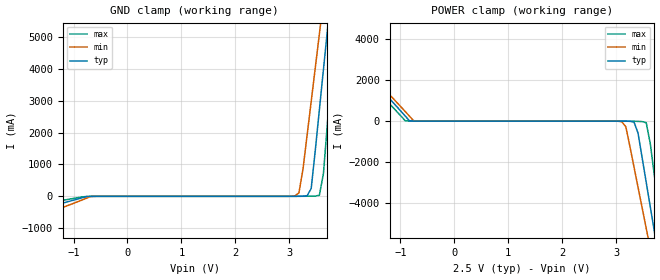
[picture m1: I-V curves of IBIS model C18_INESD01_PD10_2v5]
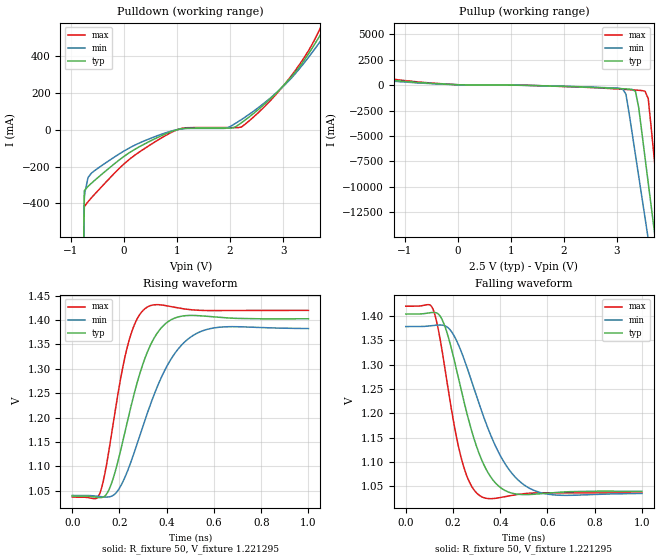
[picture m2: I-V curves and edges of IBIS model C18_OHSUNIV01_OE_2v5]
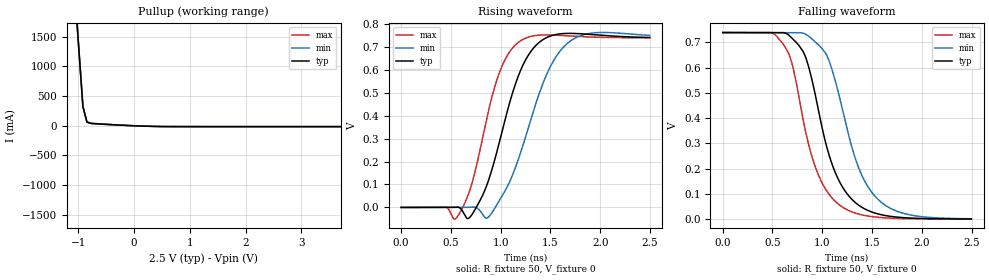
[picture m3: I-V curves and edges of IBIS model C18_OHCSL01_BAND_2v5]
|   This file is an IBIS representation of the   |
|   Integrated Device Technology, Inc.   |
|   ICS841N254I   |
|   FEMTOCLOCK NG CRYSTAL-TO-LVDS/HCSL CLOCK SYNTHESIZER   |
[IBIS Ver]   4.1
[File name]   841n254i.ibs
[File Rev]   1.0
[Date]   15 Mar 2010
[Source]   Originated at Integrated Device Technology, Inc.
[Disclaimer]
IDT hereby grants the user of this IBIS model a non-exclusive,
nontransferable license to use this IBIS model under the following terms.
Before using this IBIS model, the user should read this license.
If the user does not accept these terms,  the IBIS model should be
returned to IDT within 30 days.
   The user is granted this license only to use the IBIS model and
is not granted rights to sell, load, rent, lease or license the IBIS
model in whole or in part, or in modified form to anyone other than
user. User may modify the IBIS model to suit its specific
applications but rights to derivative works and such modifications
shall belong to IDT.
   This IBIS model is provided on an "AS IS" basis and IDT makes
absolutely no warranty with respect to the information contained
herein. IDT DISCLAIMS AND CUSTOMER WAIVES ALL WARRANTIES, EXPRESS
OR IMPLIED, INCLUDING WARRANTIES OF MERCHANTABILITY OR FITNESS FOR
A PARTICULAR PURPOSE. The entire risk as to quality and performance
is with the Customer. ACCORDINGLY, IN NO EVENT SHALL THE COMPANY BE
LIABLE FOR ANY DAMAGES, WHETHER IN CONTRACT OR TORT,INCLUDING ANY
LOST PROFITS OR OTHER INCIDENTAL, CONSEQUENTIAL, EXEMPLARY, OR
PUNITIVE DAMAGES ARISING OUT OF THE USE OR APPLICATION OF THE IBIS
model provided in this package. Further, IDT reserves the right to
make changes without notice to any product herein to improve
reliability, function, or design. IDT does not convey any license
under patent rights or any other intellectual property rights,
including those of third parties.
   IDT is not obligated to provide maintenance or support
for the licensed IBIS model.
[Copyright]   Copyright 2010 by Integrated Device Technology, Inc.
[Component]   ICS841N254KI
[Manufacturer] Integrated Device Technology, Inc.
[Package]
|LD QFN 32
|lead + wire   typ   min   max
R_pkg   72.4655m   58.886m   86.045m
L_pkg   1.47175nH   1.11650nH   1.77850nH
C_pkg   0.07747pF   0.07444pF   0.08050pF
[Pin] signal_name   model_name   R_pin   L_pin   C_pin
1   VDD   POWER   86.045m   1.77850nH   0.08050pF
2   NC   NC   76.996m   1.55783nH   0.07848pF
3   VDDA   POWER   67.941m   1.33717nH   0.07646pF
4   NC   NC   58.886m   1.11650nH   0.07444pF
5   GND   GND   58.886m   1.11650nH   0.07444pF
6   REF_CLK   C18_INESD01_PD10   67.941m   1.33717nH   0.07646pF
7   nOEA   C18_INESD01_PD10   76.996m   1.55783nH   0.07848pF
8   VDD   POWER   86.045m   1.77850nH   0.08050pF
9   nOEB   C18_INESD01_PD10   86.045m   1.77850nH   0.08050pF
10  REF_SEL   C18_INESD01_PD10   76.996m   1.55783nH   0.07848pF
11  XTAL_IN   NC   67.941m   1.33717nH   0.07646pF
12  XTAL_OUT   NC   58.886m   1.11650nH   0.07444pF
13  VDD   POWER   58.886m   1.11650nH   0.07444pF
14  BYPASS   C18_INESD01_PD10   67.941m   1.33717nH   0.07646pF
15  F_SEL0   C18_INESD01_PD10   76.996m   1.55783nH   0.07848pF
16  F_SEL1   C18_INESD01_PD10   86.045m   1.77850nH   0.08050pF
17  GND   GND   86.045m   1.77850nH   0.08050pF
18  QA1   C18_OHSUNIV01_OE   76.996m   1.55783nH   0.07848pF
19  nQA1   C18_OHSUNIV01_OE   67.941m   1.33717nH   0.07646pF
20  VDDOA   POWER   58.886m   1.11650nH   0.07444pF
21  QA0   C18_OHSUNIV01_OE   58.886m   1.11650nH   0.07444pF
22  nQA0   C18_OHSUNIV01_OE   67.941m   1.33717nH   0.07646pF
23  GND   GND   76.996m   1.55783nH   0.07848pF
24  IREF   NC   86.045m   1.77850nH   0.08050pF
25  GND   GND   86.045m   1.77850nH   0.08050pF
26  nQB1   C18_OHCSL01_BAND   76.996m   1.55783nH   0.07848pF
27  QB1   C18_OHCSL01_BAND   67.941m   1.33717nH   0.07646pF
28  VDDOB   POWER   58.886m   1.11650nH   0.07444pF
29  nQB0   C18_OHCSL01_BAND   58.886m   1.11650nH   0.07444pF
30  QB0   C18_OHCSL01_BAND   67.941m   1.33717nH   0.07646pF
31  GND   GND   76.996m   1.55783nH   0.07848pF
32  VDD   POWER   86.045m   1.77850nH   0.08050pF
[Diff Pin]  inv_pin  vdiff tdelay_typ tdelay_min  tdelay_max
18   19   NA   0   0   0
21   22   NA   0   0   0
27   26   NA   0   0   0
30   29   NA   0   0   0
[Model Selector] C18_INESD01_PD10
C18_INESD01_PD10_2v5  Buffer selection for 2v5
C18_INESD01_PD10_3v3  Buffer selection for 3v3
[Model Selector] C18_OHSUNIV01_OE
C18_OHSUNIV01_OE_2v5  Buffer selection for 2v5
C18_OHSUNIV01_OE_3v3  Buffer selection for 3v3
[Model Selector] C18_OHCSL01_BAND
C18_OHCSL01_BAND_2v5  Buffer selection for 2v5
C18_OHCSL01_BAND_3v3  Buffer selection for 3v3
| Models and submodels in the file (6): C18_INESD01_PD10_2v5 (Input), C18_OHSUNIV01_OE_2v5 (Output), C18_OHCSL01_BAND_2v5 (Open_source), C18_INESD01_PD10_3v3 (Input), C18_OHSUNIV01_OE_3v3 (Output), C18_OHCSL01_BAND_3v3 (Open_source)
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[Model] C18_INESD01_PD10_2v5
Model_type   Input
Polarity   Non-Inverting
Vinl = 0.7V
Vinh = 1.7V
|   typ   min   max
C_comp   2pF   1.5pF   2.5pF
|   typ   min   max
[Voltage range]   2.5V   2.375V   2.625V
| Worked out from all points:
|   GND clamp passes 1 mA (typ) near -0.63 V on its own axis
|   POWER clamp passes 1 mA (typ) near -0.64 V on its own axis
[GND_clamp]
|Voltage   I (typ)   I (min)   I (max)
-2.5V     -750.5mA   -1.114A    -470.1mA
-681.8mV  -2.012mA   -6.108mA   -2.703mA
3.106V    574.9uA    12.03mA    60.91uA
3.182V    1.627mA    109.8mA    268.6uA
3.258V    3.996mA    865.2mA    1.08mA
3.409V    245.5mA    2.979A     5.107mA
3.561V    2.713A     5.094A     32.39mA
3.636V    3.983A     6.152A     713.8mA
3.712V    5.254A     7.21A      2.338A
3.788V    6.512A     8.257A     3.947A
3.864V    7.757A     9.294A     5.539A
5V        25.01A     23.66A     27.6A
[Power_clamp]
|Voltage   I (typ)   I (min)   I (max)
-2.5V     4.507A     4.598A     4.173A
-833.3mV  19.22mA    247mA      7.107mA
-681.8mV  1.627mA    3.397mA    2.058mA
3.106V    -505.4uA   -25.77mA   -25.85uA
3.182V    -2.012mA   -269.5mA   -184.8uA
3.333V    -42.94mA   -2.236A    -4.112mA
3.409V    -586.1mA   -3.238A    -10.29mA
3.561V    -2.995A    -5.243A    -78.7mA
3.636V    -4.2A      -6.246A    -1.114A
3.712V    -5.406A    -7.249A    -2.656A
3.864V    -7.781A    -9.225A    -5.693A
5V        -24.15A    -22.85A    -26.63A
[Model] C18_OHSUNIV01_OE_2v5
Model_type   Output
Polarity   Non-Inverting
|   typ   min   max
C_comp   2pF   1.5pF   2.5pF
Vmeas = 1.22V
Rref = 50
Cref = 0
Vref = 1.22V
|   typ   min   max
[Voltage range]   2.5V   2.375V   2.625V
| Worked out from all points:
|   slope of the pulldown table from 0 to 0.375 V, typ, clamps not added: 5.71 ohm
|   slope of the pullup table from 0 to 0.375 V, typ, clamps not added: 13.8 ohm
|   rising waveform, R_fixture 50, V_fixture 1.221295: 20-80 % time 120ps typ, 163ps min, 83.5ps max; typ from 1.04 V to 1.4 V
|   falling waveform, R_fixture 50, V_fixture 1.221295: 20-80 % time 120ps typ, 163ps min, 83.5ps max; typ from 1.4 V to 1.04 V
[Pulldown]
|Voltage   I (typ)   I (min)   I (max)
-2.5V     -67.43A    -58.92A    -81.85A
-1.1V     -9.702A    -10.9A     -7.965A
-750mV    -331.8mA   -375mA     -418.1mA
-679.8mV  -308.2mA   -260mA     -391.8mA
-137.7mV  -174.7mA   -139.8mA   -223.4mA
1.007V    1.311mA    1.573mA    780.8uA
1.91V     9.611mA    8.297mA    12.19mA
2.211V    38.17mA    55.54mA    15.12mA
3.054V    256.3mA    251.4mA    257.4mA
3.717V    524.8mA    488.3mA    563.9mA
3.898V    615.6mA    567.2mA    679mA
5V        5.426A     6.175A     4.372A
[Pullup]
|Voltage   I (typ)   I (min)   I (max)
-2.5V     5.425A     5.436A     5.512A
-2.15V    2.951A     3.381A     2.337A
-1.8V     849.6mA    1.334A     1.044A
-1.45V    590.8mA    482.1mA    748.7mA
3.115V    -358.2mA   -400.5mA   -410mA
3.175V    -374mA     -882.6mA   -428.2mA
3.356V    -626.9mA   -6.875A    -487.4mA
3.536V    -7.145A    -13.06A    -599.5mA
3.597V    -9.622A    -15.12A    -1.338A
3.717V    -14.58A    -19.25A    -7.616A
3.837V    -19.53A    -23.38A    -13.95A
5V        -67.44A    -63.23A    -75.24A
[Ramp]
|   typ   min   max
dV/dt_r   0.299/0.186n   0.279/0.25n   0.318/0.131n
dV/dt_f   0.299/0.186n   0.279/0.25n   0.318/0.131n
R_load =   50.0000
[Rising Waveform]
R_fixture = 50
V_fixture   =1.221295   |Vcc_typ
V_fixture_min=1.209005  |Vcc_min
V_fixture_max=1.22817  |Vcc_max
C_fixture = 0.0p
| Time   typ   min   max
0s        1.039V     1.04V      1.037V
117.1ps   1.036V     1.038V     1.045V
165.2ps   1.063V     1.038V     1.162V
230.2ps   1.185V     1.086V     1.339V
266.3ps   1.256V     1.134V     1.394V
308.3ps   1.322V     1.195V     1.424V
395.4ps   1.393V     1.3V       1.43V
520.5ps   1.409V     1.371V     1.421V
645.6ps   1.405V     1.386V     1.419V
1ns       1.403V     1.383V     1.42V
[Falling Waveform]
R_fixture = 50
V_fixture   =1.221295   |Vcc_typ
V_fixture_min=1.209005  |Vcc_min
V_fixture_max=1.22817  |Vcc_max
C_fixture = 0.0p
| Time   typ   min   max
0s        1.404V     1.378V     1.42V
117.1ps   1.407V     1.38V      1.412V
165.2ps   1.379V     1.38V      1.294V
230.2ps   1.257V     1.332V     1.117V
266.3ps   1.186V     1.284V     1.062V
308.3ps   1.12V      1.223V     1.033V
395.4ps   1.05V      1.118V     1.027V
520.5ps   1.033V     1.047V     1.036V
645.6ps   1.038V     1.032V     1.037V
1ns       1.04V      1.035V     1.036V
[Model] C18_OHCSL01_BAND_2v5
Model_type   Open_source
Polarity   Non-Inverting
|   typ   min   max
C_comp   2pF   1.5pF   2.5pF
Vmeas = 0.33V
Rref = 50
Cref = 0
Vref = 0V
|   typ   min   max
[Voltage range]   2.5V   2.375V   2.625V
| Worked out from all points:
|   slope of the pullup table from 0 to 0.375 V, typ, clamps not added: 33.5 ohm
|   rising waveform, R_fixture 50, V_fixture 0: 20-80 % time 295ps typ, 356ps min, 253ps max; typ from 0 V to 0.74 V
|   falling waveform, R_fixture 50, V_fixture 0: 20-80 % time 302ps typ, 330ps min, 282ps max; typ from 0.738 V to 0 V
[Pullup]
|Voltage   I (typ)   I (min)   I (max)
-2.5V     21.73A     21.71A     21.74A
-1.06V    2.243A     2.239A     2.248A
-987.9mV  1.276A     1.272A     1.28A
-916.2mV  324mA      320.3mA    327.6mA
-844.5mV  62.93mA    59.54mA    66.21mA
-772.8mV  40.5mA     37.42mA    43.47mA
374.8mV   -11.19mA   -10.62mA   -11.67mA
4.104V    -32.38mA   -28.13mA   -39.79mA
4.176V    -185.1mA   -178.9mA   -194.6mA
4.248V    -1.05A     -1.042A    -1.061A
4.32V     -1.996A    -1.987A    -2.009A
5V        -10.99A    -10.96A    -11.01A
[Ramp]
|   typ   min   max
dV/dt_r   0.645/0.505n   0.646/0.604n   0.641/0.43n
dV/dt_f   0.59/0.502n   0.589/0.549n   0.59/0.47n
R_load =   50.0000
[Rising Waveform]
R_fixture = 50
V_fixture = 0   | VCC_typ
V_fixture_max = 0   | VCC_max
V_fixture_min = 0   | VCC_min
C_fixture = 0.0p
| Time   typ   min   max
0s        451.1pV    473.2pV    430.3pV
447.9ps   -29.29uV   324.8nV    1.138mV
540.5ps   1.037mV    6.718uV    -50.27mV
693.2ps   -41.84mV   877.5uV    78.5mV
858.4ps   93.67mV    -46.65mV   383.3mV
968.5ps   252.6mV    16.73mV    563.3mV
1.194ns   590mV      230mV      723.8mV
1.449ns   736.7mV    565.8mV    751.2mV
1.657ns   757.8mV    709mV      747.5mV
2.498ns   740mV      748.9mV    738.7mV
[Falling Waveform]
R_fixture = 50
V_fixture = 0   | VCC_typ
V_fixture_max = 0   | VCC_max
V_fixture_min = 0   | VCC_min
C_fixture = 0.0p
| Time   typ   min   max
0s        738.4mV    738.1mV    738.7mV
523ps     738.1mV    738.1mV    730.7mV
668.2ps   726.7mV    737.8mV    650.1mV
765.8ps   687mV      738.2mV    483.8mV
940.9ps   471.3mV    697.6mV    195.2mV
1.059ns   266.8mV    636.7mV    103.7mV
1.176ns   146mV      478.3mV    54.92mV
1.361ns   56.44mV    207.6mV    20.24mV
1.572ns   19.35mV    73.87mV    6.702mV
2.498ns   478.4uV    1.297mV    238.8uV
